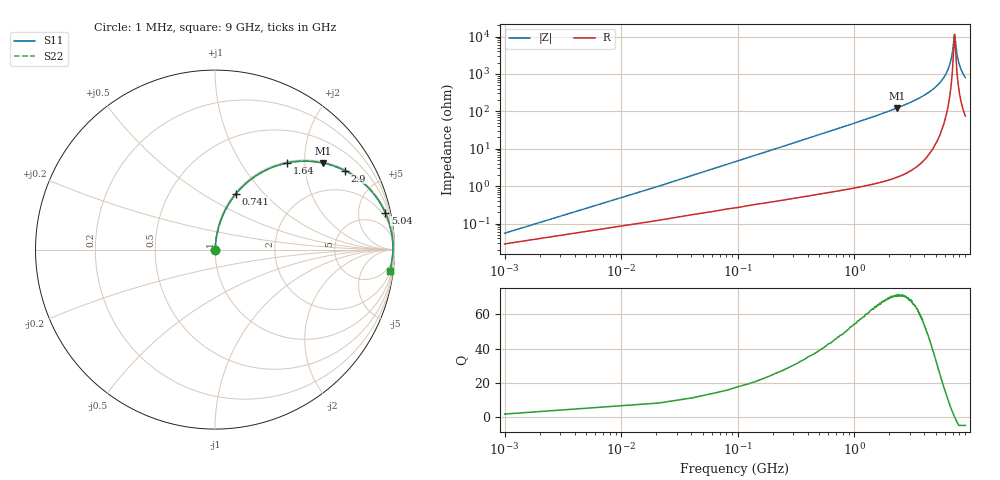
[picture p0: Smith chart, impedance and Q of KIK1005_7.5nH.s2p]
!version-3
!date-01.2023
!Series
# MHz S RI R 50
!Freq ReS11 ImS11 ReS21 ImS21 ReS12 ImS12 ReS22 ImS22
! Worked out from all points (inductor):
!   451 points, 1 MHz to 9 GHz, reference 50 ohm
!   read as one part in series: L = 7.5 nH near 41 MHz
!   highest Q = 71.1 at 2.34 GHz (marker M1), where L = 8.37 nH
!   self-resonance near 7.26 GHz
!   S11 on the Smith chart (normalised r, x): 1 MHz: 1.00, +0.00; 741 MHz: 1.02, +0.71; 1.64 GHz: 1.02, +1.63; 2.9 GHz: 1.05, +3.25; 5.04 GHz: 1.28, +9.15; 9 GHz: 2, -16
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1  0.00027 0.000471  0.9997 -0.000471  0.9997 -0.000471  0.00027 0.000471
61  0.00292 0.0286  0.9971 -0.0286  0.9971 -0.0286  0.00292 0.0286
101  0.00495 0.0472  0.9951 -0.0472  0.9951 -0.0472  0.00495 0.0472
141  0.00755 0.0658  0.9924 -0.0658  0.9924 -0.0658  0.00755 0.0658
361  0.033 0.1641  0.967 -0.1641  0.967 -0.1641  0.033 0.1641
741  0.1159 0.3096  0.8841 -0.3096  0.8841 -0.3096  0.1159 0.3096
1520  0.3619 0.4728  0.6381 -0.4728  0.6381 -0.4728  0.3619 0.4728
1640  0.4006 0.4825  0.5994 -0.4825  0.5994 -0.4825  0.4006 0.4825
2340  0.6011 0.4827  0.3989 -0.4827  0.3989 -0.4827  0.6011 0.4827
2900  0.7228 0.4405  0.2772 -0.4405  0.2772 -0.4405  0.7228 0.4405
3020  0.7445 0.4289  0.2555 -0.4289  0.2555 -0.4289  0.7445 0.4289
4520  0.9184 0.2624  0.0816 -0.2624  0.0816 -0.2624  0.9184 0.2624
5040  0.9487 0.2058  0.0513 -0.2058  0.0513 -0.2058  0.9487 0.2058
6020  0.981 0.1076  0.019 -0.1076  0.019 -0.1076  0.981 0.1076
6780  0.9903 0.0397  0.00966 -0.0397  0.00966 -0.0397  0.9903 0.0397
7000  0.9912 0.0214  0.00882 -0.0214  0.00882 -0.0214  0.9912 0.0214
7240  0.9913 0.00206  0.0087 -0.00206  0.0087 -0.00206  0.9913 0.00206
7320  0.9912 -0.00424  0.00883 0.00424  0.00883 0.00424  0.9912 -0.00424
7520  0.9905 -0.0197  0.0095 0.0197  0.0095 0.0197  0.9905 -0.0197
7740  0.9892 -0.0362  0.0108 0.0362  0.0108 0.0362  0.9892 -0.0362
8060  0.9864 -0.0592  0.0135 0.0592  0.0135 0.0592  0.9864 -0.0592
9000  0.9732 -0.1209  0.0268 0.1209  0.0268 0.1209  0.9732 -0.1209
